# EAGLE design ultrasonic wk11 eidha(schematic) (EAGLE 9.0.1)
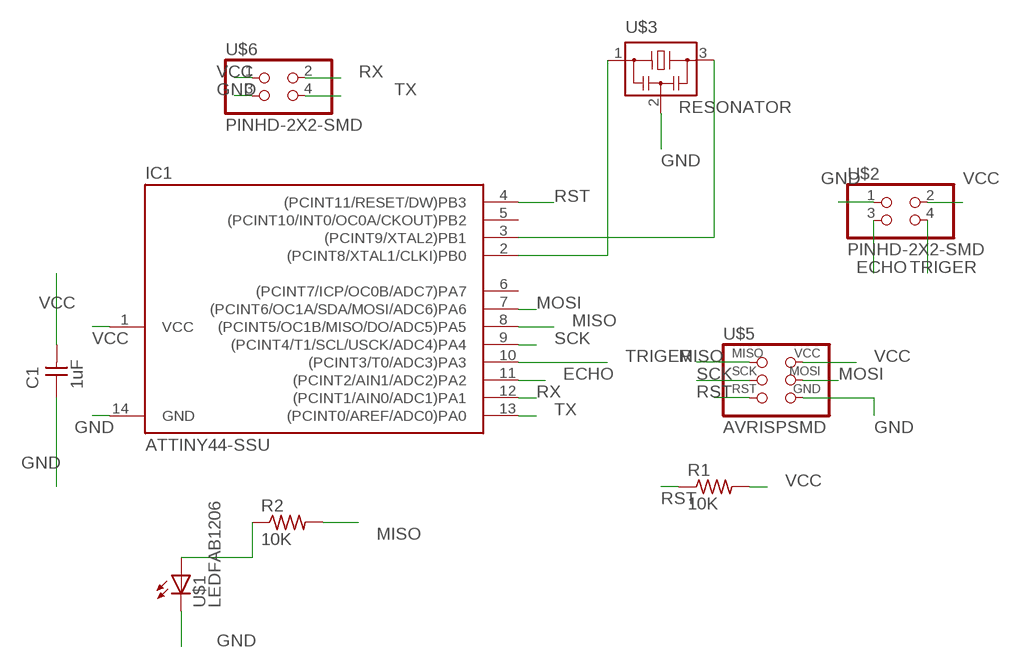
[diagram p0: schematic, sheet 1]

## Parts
C1  1uF  CAP-UNPOLARIZEDFAB  [C1206FAB]
IC1  ATTINY44-SSU  [SOIC14]
R1  10K  RES-US1206FAB  [R1206FAB]
R2  10K  RES-US1206FAB  [R1206FAB]
U$1  LEDFAB1206  [LED1206FAB]
U$2  PINHD-2X2-SMD  [2X02SMD]
U$3  RESONATOR  [EFOBM]
U$5  AVRISPSMD  [2X03SMD]
U$6  PINHD-2X2-SMD  [2X02SMD]

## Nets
ECHO: IC1.11((PCINT2/AIN1/ADC2)PA2) U$2.3
GND: C1.1 IC1.14(GND) U$1.2(C) U$2.1 U$3.2 U$5.6(GND) U$6.3
MISO: IC1.8((PCINT5/OC1B/MISO/DO/ADC5)PA5) R2.2 U$5.1(MISO)
MOSI: IC1.7((PCINT6/OC1A/SDA/MOSI/ADC6)PA6) U$5.4(MOSI)
N$1: R2.1 U$1.1(A)
N$3: IC1.2((PCINT8/XTAL1/CLKI)PB0) U$3.1
N$8: IC1.3((PCINT9/XTAL2)PB1) U$3.3
RST: IC1.4((PCINT11/RESET/DW)PB3) R1.1 U$5.5(RST)
RX: IC1.12((PCINT1/AIN0/ADC1)PA1) U$6.2
SCK: IC1.9((PCINT4/T1/SCL/USCK/ADC4)PA4) U$5.3(SCK)
TRIGER: IC1.10((PCINT3/T0/ADC3)PA3) U$2.4
TX: IC1.13((PCINT0/AREF/ADC0)PA0) U$6.4
VCC: C1.2 IC1.1(VCC) R1.2 U$2.2 U$5.2(VCC) U$6.1
Unconnected: IC1.5((PCINT10/INT0/OC0A/CKOUT)PB2) IC1.6((PCINT7/ICP/OC0B/ADC7)PA7)

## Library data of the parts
C1 = fab:CAP-UNPOLARIZED
IC1 = fab:ATTINY44
R1 R2 = fab:RES-US: Resistor (US Symbol)
U$1 = fab:LED: LED
U$2 U$6 = fab:PINHD-2X2-SMD
U$3 = fab:RESONATOR
U$5 = fab:AVRISP

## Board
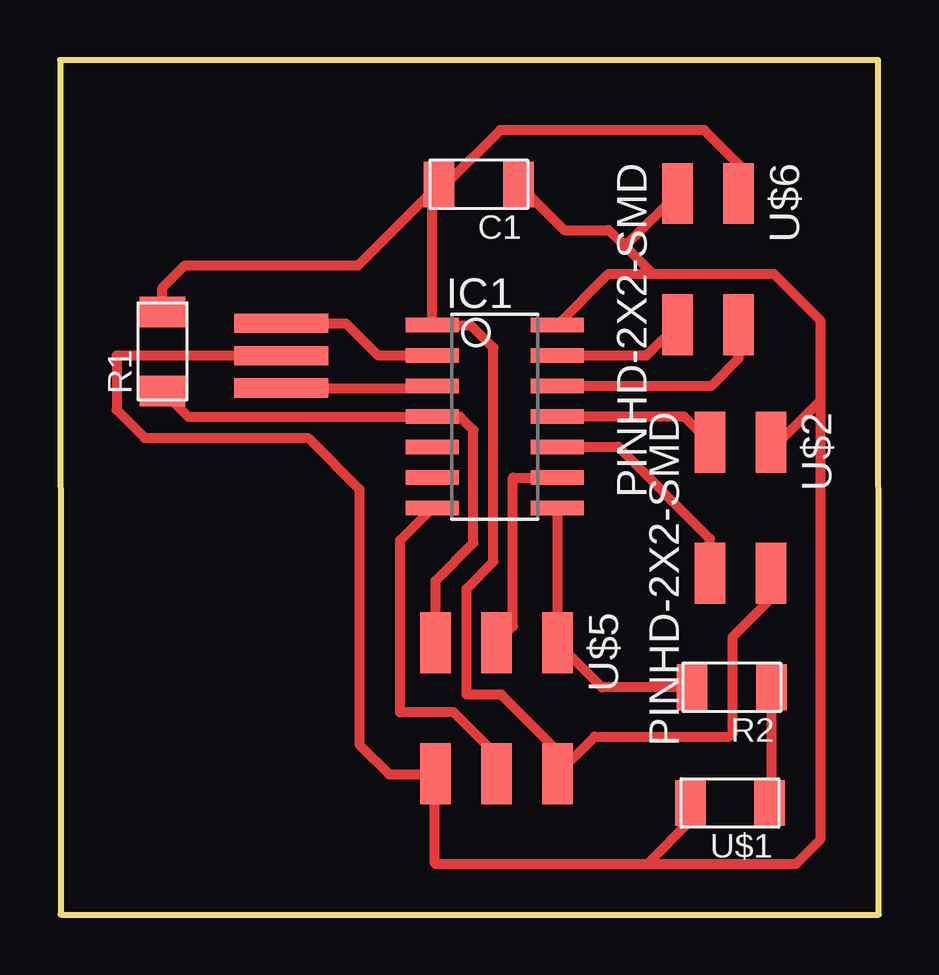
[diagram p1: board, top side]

Size 34.12 x 35.61 mm. Coordinates in mm from the lower left corner, seen from the top.
Outline: 0.03,0 34.12,0 34.09,35.61 0,35.61 0.03,0
Copper layers (1*16): Top 0.035mm / dielectric 1.5mm / Bottom 0.035mm
Design rules "default *": minimum track width 6mil, minimum drill 0.35mm, track to track 16mil, track to pad 16mil, pad to pad 16mil, via to via 16mil, smd to smd 6mil, copper to edge 40mil, drill to drill 6mil, minimum pad ring 10mil, minimum via ring 8mil, stop-mask expansion 4mil, vias tented up to drill 0mil, thermal gap 10mil

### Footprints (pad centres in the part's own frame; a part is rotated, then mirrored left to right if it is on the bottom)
C1206FAB = smd 1.27 x 1.905: 1 -1.651,0; 2 1.651,0
SOIC14 = smd 0.61 x 2.21: 1 -3.81,-2.603; 2 -2.54,-2.603; 3 -1.27,-2.603; 4 0,-2.603; 5 1.27,-2.603; 6 2.54,-2.603; 7 3.81,-2.603; 8 3.81,2.603; 9 2.54,2.603; 10 1.27,2.603; 11 0,2.603; 12 -1.27,2.603; 13 -2.54,2.603; 14 -3.81,2.603
R1206FAB = smd 1.27 x 1.905: 1 -1.651,0; 2 1.651,0
LED1206FAB = smd 1.27 x 1.905: 1 -1.651,0; 2 1.651,0
2X02SMD = smd 2.54 x 1.27: 1 -2.54,1.27; 2 2.92,1.27; 3 -2.54,-1.27; 4 2.92,-1.27
EFOBM = smd 0.8 x 3.9: 1 -1.35,0; 2 0,0; 3 1.35,0
2X03SMD = smd 2.54 x 1.27: 1 -2.54,2.54; 2 2.92,2.54; 3 -2.54,0; 4 2.92,0; 5 -2.54,-2.54; 6 2.92,-2.54

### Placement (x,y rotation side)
C1  17.45,30.43 180 top
IC1  18.11,20.75 270 top
R1  4.27,23.47 90 top
R2  27.99,9.47 180 top
U$1  27.91,4.65 180 top
U$2  28.35,17.15 270 top
U$3  9.22,23.29 270 top
U$5  18.19,8.79 270 top
U$6  27,27.51 270 top

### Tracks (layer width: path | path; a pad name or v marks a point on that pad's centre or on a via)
ECHO
  Top 0.406: U$2.3 26.01,20.75 IC1.11
GND
  Top 0.406: IC1.14 22.85,26.7 24.69,26.7 | 31.67,21.41 31.67,24.76 29.74,26.7 24.69,26.7 | 31.67,21.41 31.67,3.12 30.66,2.11 24.46,2.11 | 24.46,2.11 15.65,2.11 15.62,2.13 15.62,5.84 | 15.62,5.84 U$5.6 | C1.1 21.01,28.52 22.86,28.52 23.42,27.97 | 23.42,27.97 24.69,26.7 | U$6.3 23.65,27.97 23.42,27.97 | 31.67,21.41 29.95,19.68 U$2.1 | U$1.2 26.26,3.91 24.46,2.11 | U$3.2 2.36,23.29 2.36,21.03 3.53,19.86 10.34,19.86 12.47,17.73 12.47,7.09 13.72,5.84 15.62,5.84
MISO
  Top 0.406: IC1.8 20.71,11.34 U$5.1 22.58,9.47 R2.2
MOSI
  Top 0.406: U$5.4 18.19,6.65 16.41,8.43 14.17,8.43 14.17,15.61 IC1.7
N$1
  Top 0.406: R2.1 29.64,5.16 U$1.1
N$3
  Top 0.406: U$3.1 11.91,24.64 13.23,23.32 15.48,23.32 IC1.2
N$8
  Top 0.406: U$3.3 15.43,21.94 IC1.3
RST
  Top 0.406: U$5.5 15.65,13.92 17.22,15.49 17.22,20.19 16.66,20.75 IC1.4 5.33,20.75 R1.1
RX
  Top 0.406: U$6.2 28.27,23.16 27.13,22.02 IC1.12
SCK
  Top 0.406: U$5.3 18.87,12.01 18.87,18.21 IC1.9
TRIGER
  Top 0.406: U$2.4 27.08,15.67 23.24,19.51 23.22,19.48 IC1.10
TX
  Top 0.406: U$6.4 24.43,23.29 IC1.13
VCC
  Top 0.406: R1.2 4.27,26.11 5.21,27.05 12.42,27.05 C1.2 | C1.2 15.51,30.14 IC1.1 15.53,24.54 17.15,24.54 18.06,23.62 18.06,14.71 16.94,13.59 16.94,9.17 18.39,9.17 20.73,6.83 U$5.2 | U$5.2 22.28,7.42 27.89,7.42 28.04,7.57 28.04,11.58 29.62,13.16 U$2.2 | U$6.1 28.27,31.27 26.85,32.69 18.34,32.69 16.08,30.43 C1.2 | U$5.2 20.73,6.38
